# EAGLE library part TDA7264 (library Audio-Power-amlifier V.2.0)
The TDA7264 is class AB dual Audio power amplifier assembled in the Multiwatt package, specially designed for high quality sound application as Hi-Fi music centers and stereo TV sets.
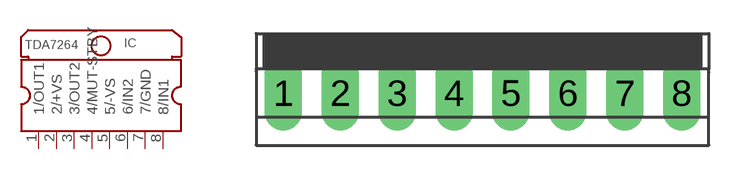
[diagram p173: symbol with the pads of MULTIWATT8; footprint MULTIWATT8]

Designator prefix IC

## TDA7264  [MULTIWATT8]
1  1/OUT1  out
2  2/+VS  pwr
3  3/OUT2  out
4  4/MUT-STBY  in
5  5/-VS  pwr
6  6/IN2  in
7  7/GND  pwr
8  8/IN1  in

## Footprint MULTIWATT8 (pad centres in mm)
drill 0.8 pad 1.676 long: 1 -8.89,0; 2 -6.35,0; 3 -3.81,0; 4 -1.27,0; 5 1.27,0; 6 3.81,0; 7 6.35,0; 8 8.89,0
